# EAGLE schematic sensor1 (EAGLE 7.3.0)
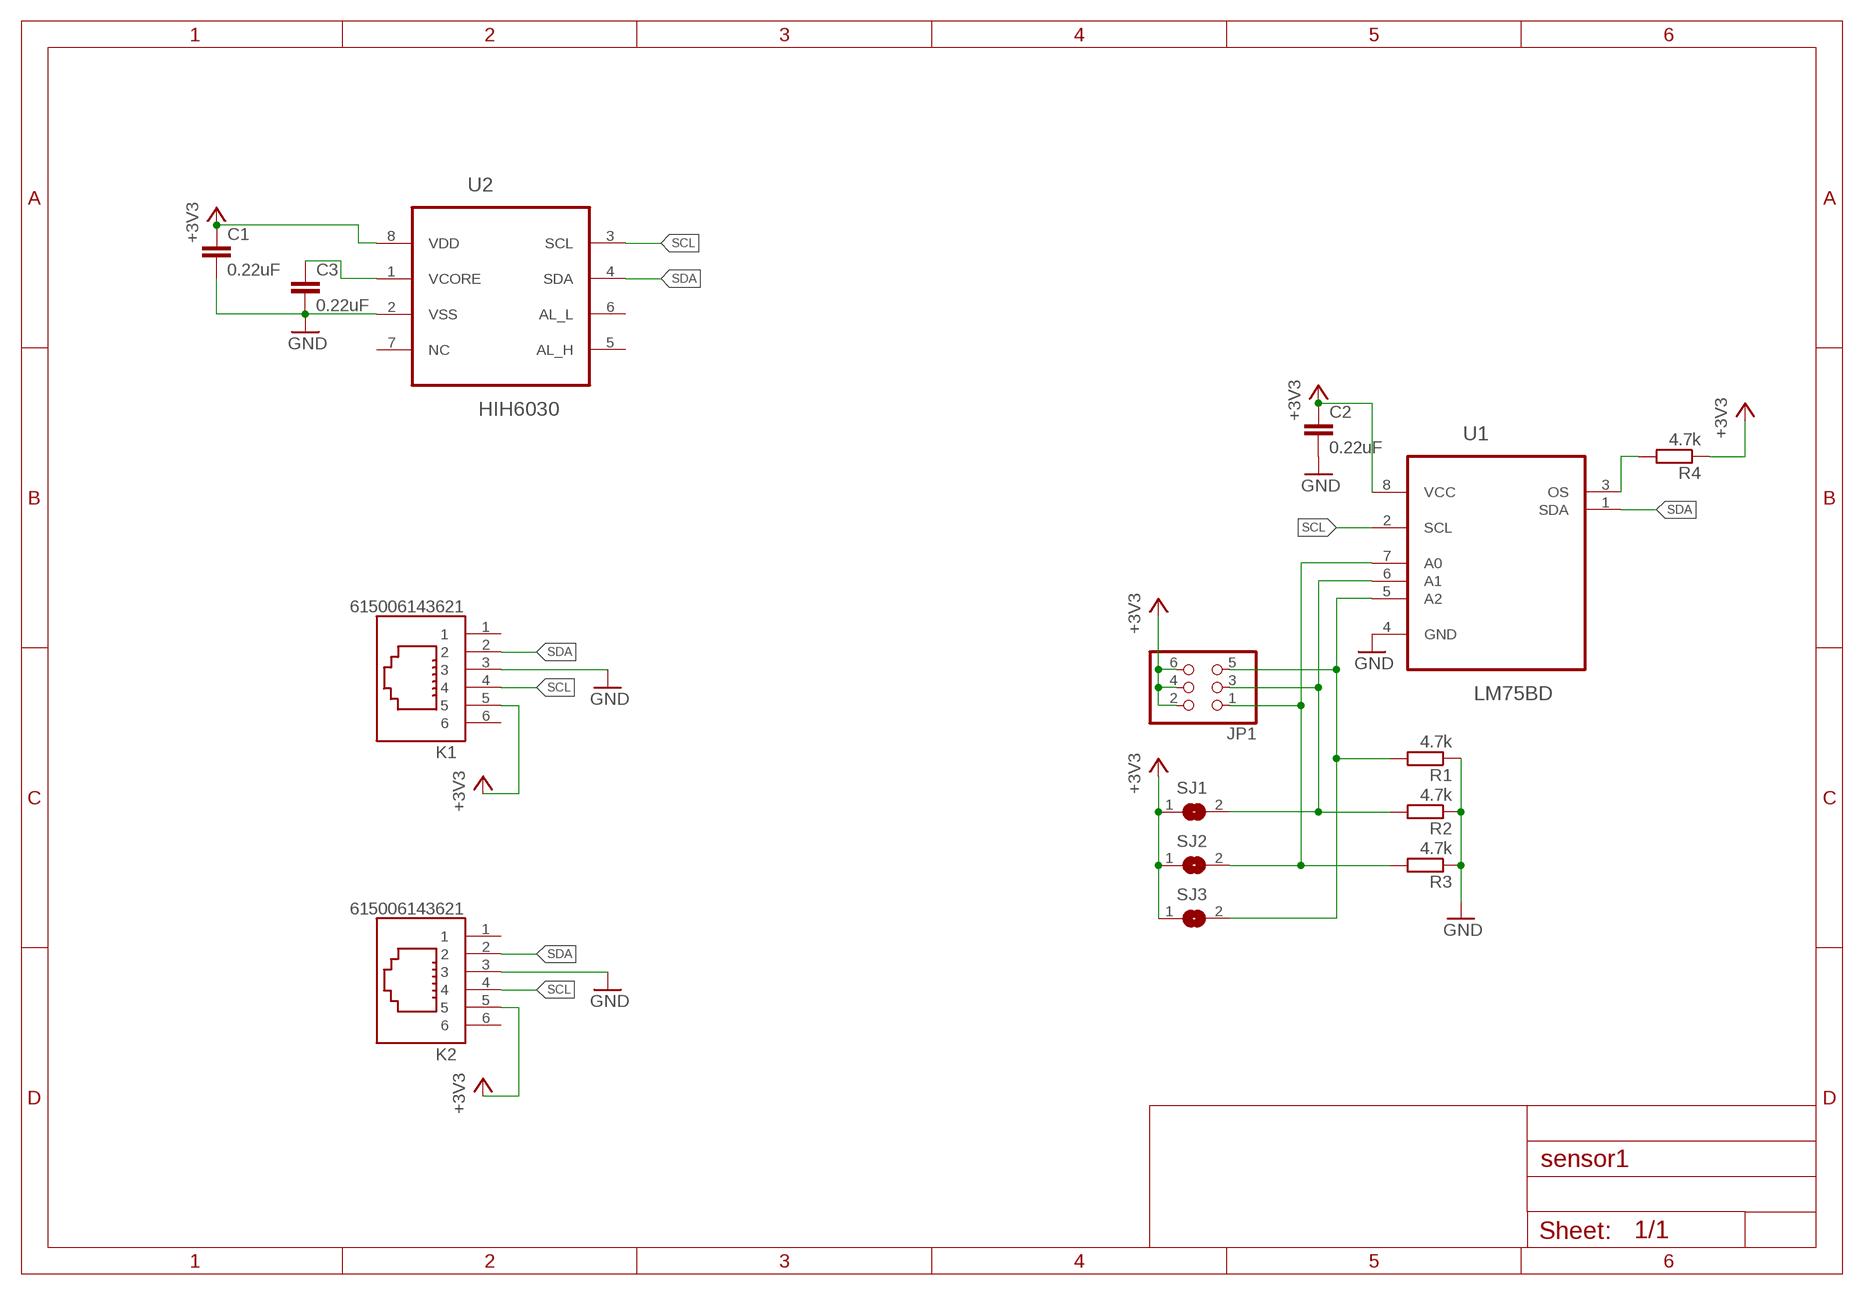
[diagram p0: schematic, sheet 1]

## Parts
C1  0.22uF  C-EUC0805  [C0805]
C2  0.22uF  C-EUC0805  [C0805]
C3  0.22uF  C-EUC0805  [C0805]
JP1  PINHD-2X3/90  [2X03/90]
K1  615006143621  [615006143621]
K2  615006143621  [615006143621]
R1  4.7k  R-EU_R0805  [R0805]
R2  4.7k  R-EU_R0805  [R0805]
R3  4.7k  R-EU_R0805  [R0805]
R4  4.7k  R-EU_R0805  [R0805]
SJ1  SJ  [SJ]
SJ2  SJ  [SJ]
SJ3  SJ  [SJ]
U1  LM75BD  [SOIC127P600X175-8N]
U2  HIH6030  [SOIC127P600X175-8N]

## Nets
+3V3: C1.1 C2.1 JP1.2 JP1.4 JP1.6 K1.5 K2.5 R4.1 SJ1.1 SJ2.1 SJ3.1 U1.8(VCC) U2.8(VDD)
GND: C1.2 C2.2 C3.2 K1.3 K2.3 R1.1 R2.1 R3.1 U1.4(GND) U2.2(VSS)
N$1: JP1.3 R2.2 SJ1.2 U1.6(A1)
N$2: JP1.1 R3.2 SJ2.2 U1.7(A0)
N$4: C3.1 U2.1(VCORE)
N$7: R4.2 U1.3(OS)
N$8: JP1.5 R1.2 SJ3.2 U1.5(A2)
SCL: K1.4 K2.4 U1.2(SCL) U2.3(SCL)
SDA: K1.2 K2.2 U1.1(SDA) U2.4(SDA)
Unconnected: K1.1 K1.6 K2.1 K2.6 U2.5(AL_H) U2.6(AL_L) U2.7(NC)

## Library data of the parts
C1-C3 = rcl:C-EU: CAPACITOR, European symbol
JP1 = pinhead:PINHD-2X3: PIN HEADER
K1 K2 = ModularJackliegendungeschirmtWR-MJ:615006143621: WR-MJ Horizontal Plastic 6P6C Modular Jack Tab Down, 6 Pins=>Code : Con_I-O_MJ-H_Plastic_Down_615006143621 Details see: http://katalog.we-online.de/en/em/615_006_143_621 Created 2014-07-10, Karrer Zheng 2014 (C) Würth Elektronik
R1-R4 = rcl:R-EU_: RESISTOR, European symbol
SJ1-SJ3 = jumper:SJ: SMD solder JUMPER
U1 = NXP_By_element14_Batch_1:LM75BD: Digital temperature sensor and thermal watchdog; MPN: LM75BD; OC_FARNELL: 1854077; OC_NEWARK: 39T1312; PACKAGE: SO-8; SUPPLIER: NXP
U2 = hih6030:HIH6030: Digital temperature sensor and thermal watchdog; PACKAGE: SO-8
